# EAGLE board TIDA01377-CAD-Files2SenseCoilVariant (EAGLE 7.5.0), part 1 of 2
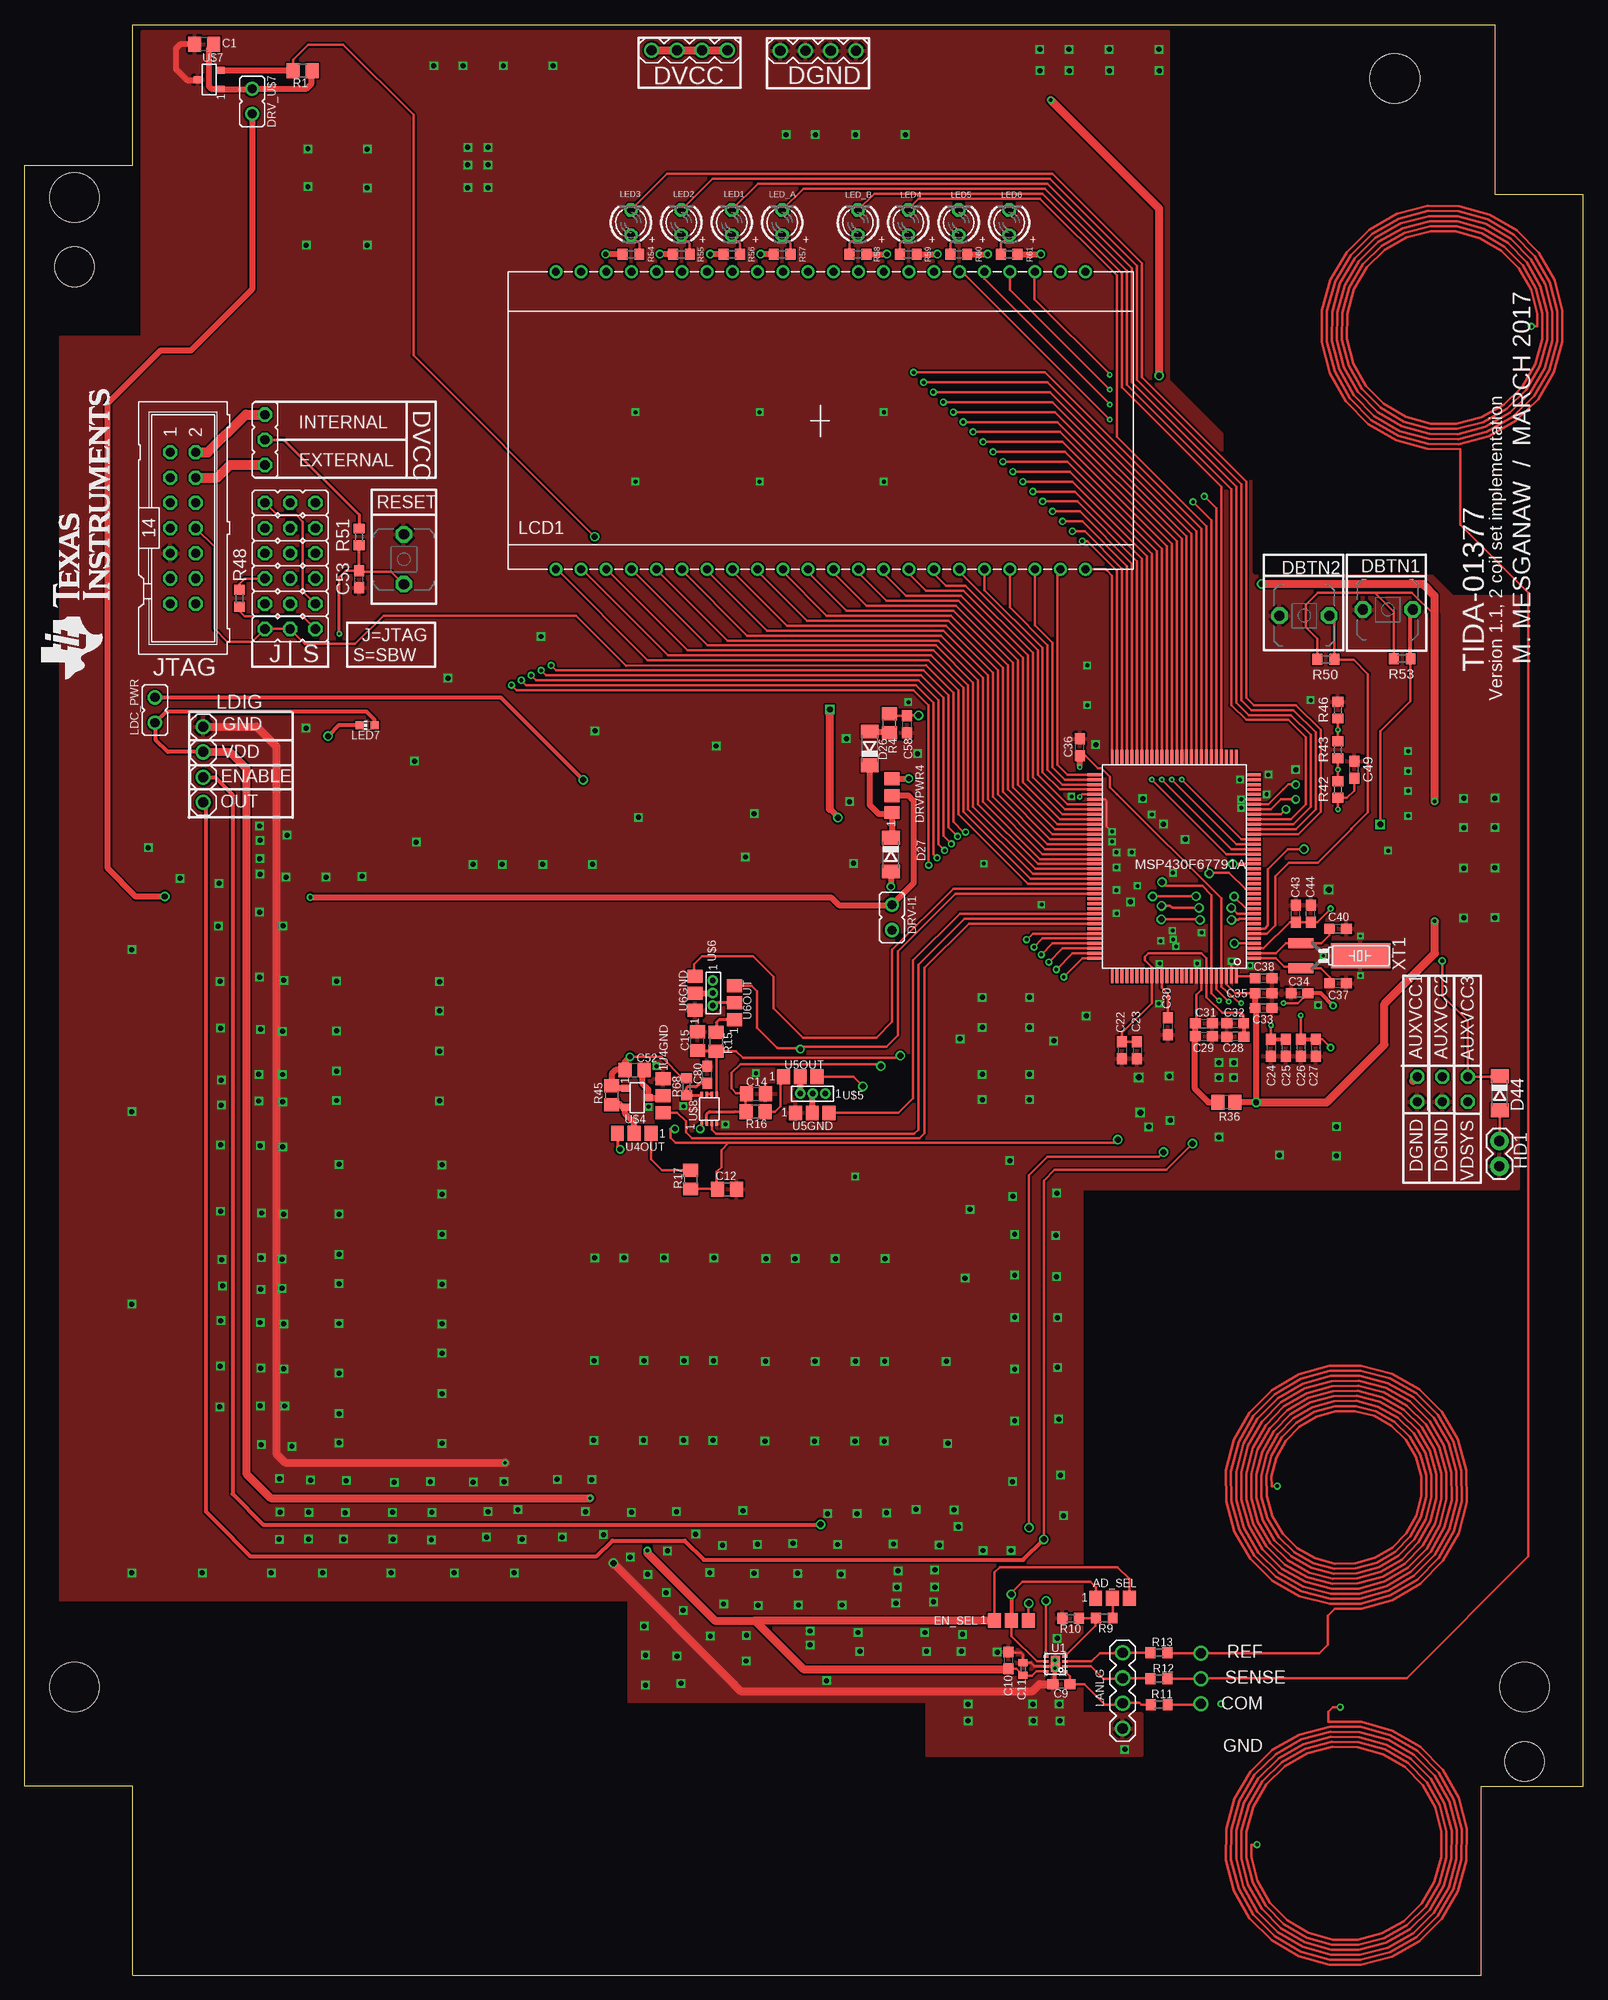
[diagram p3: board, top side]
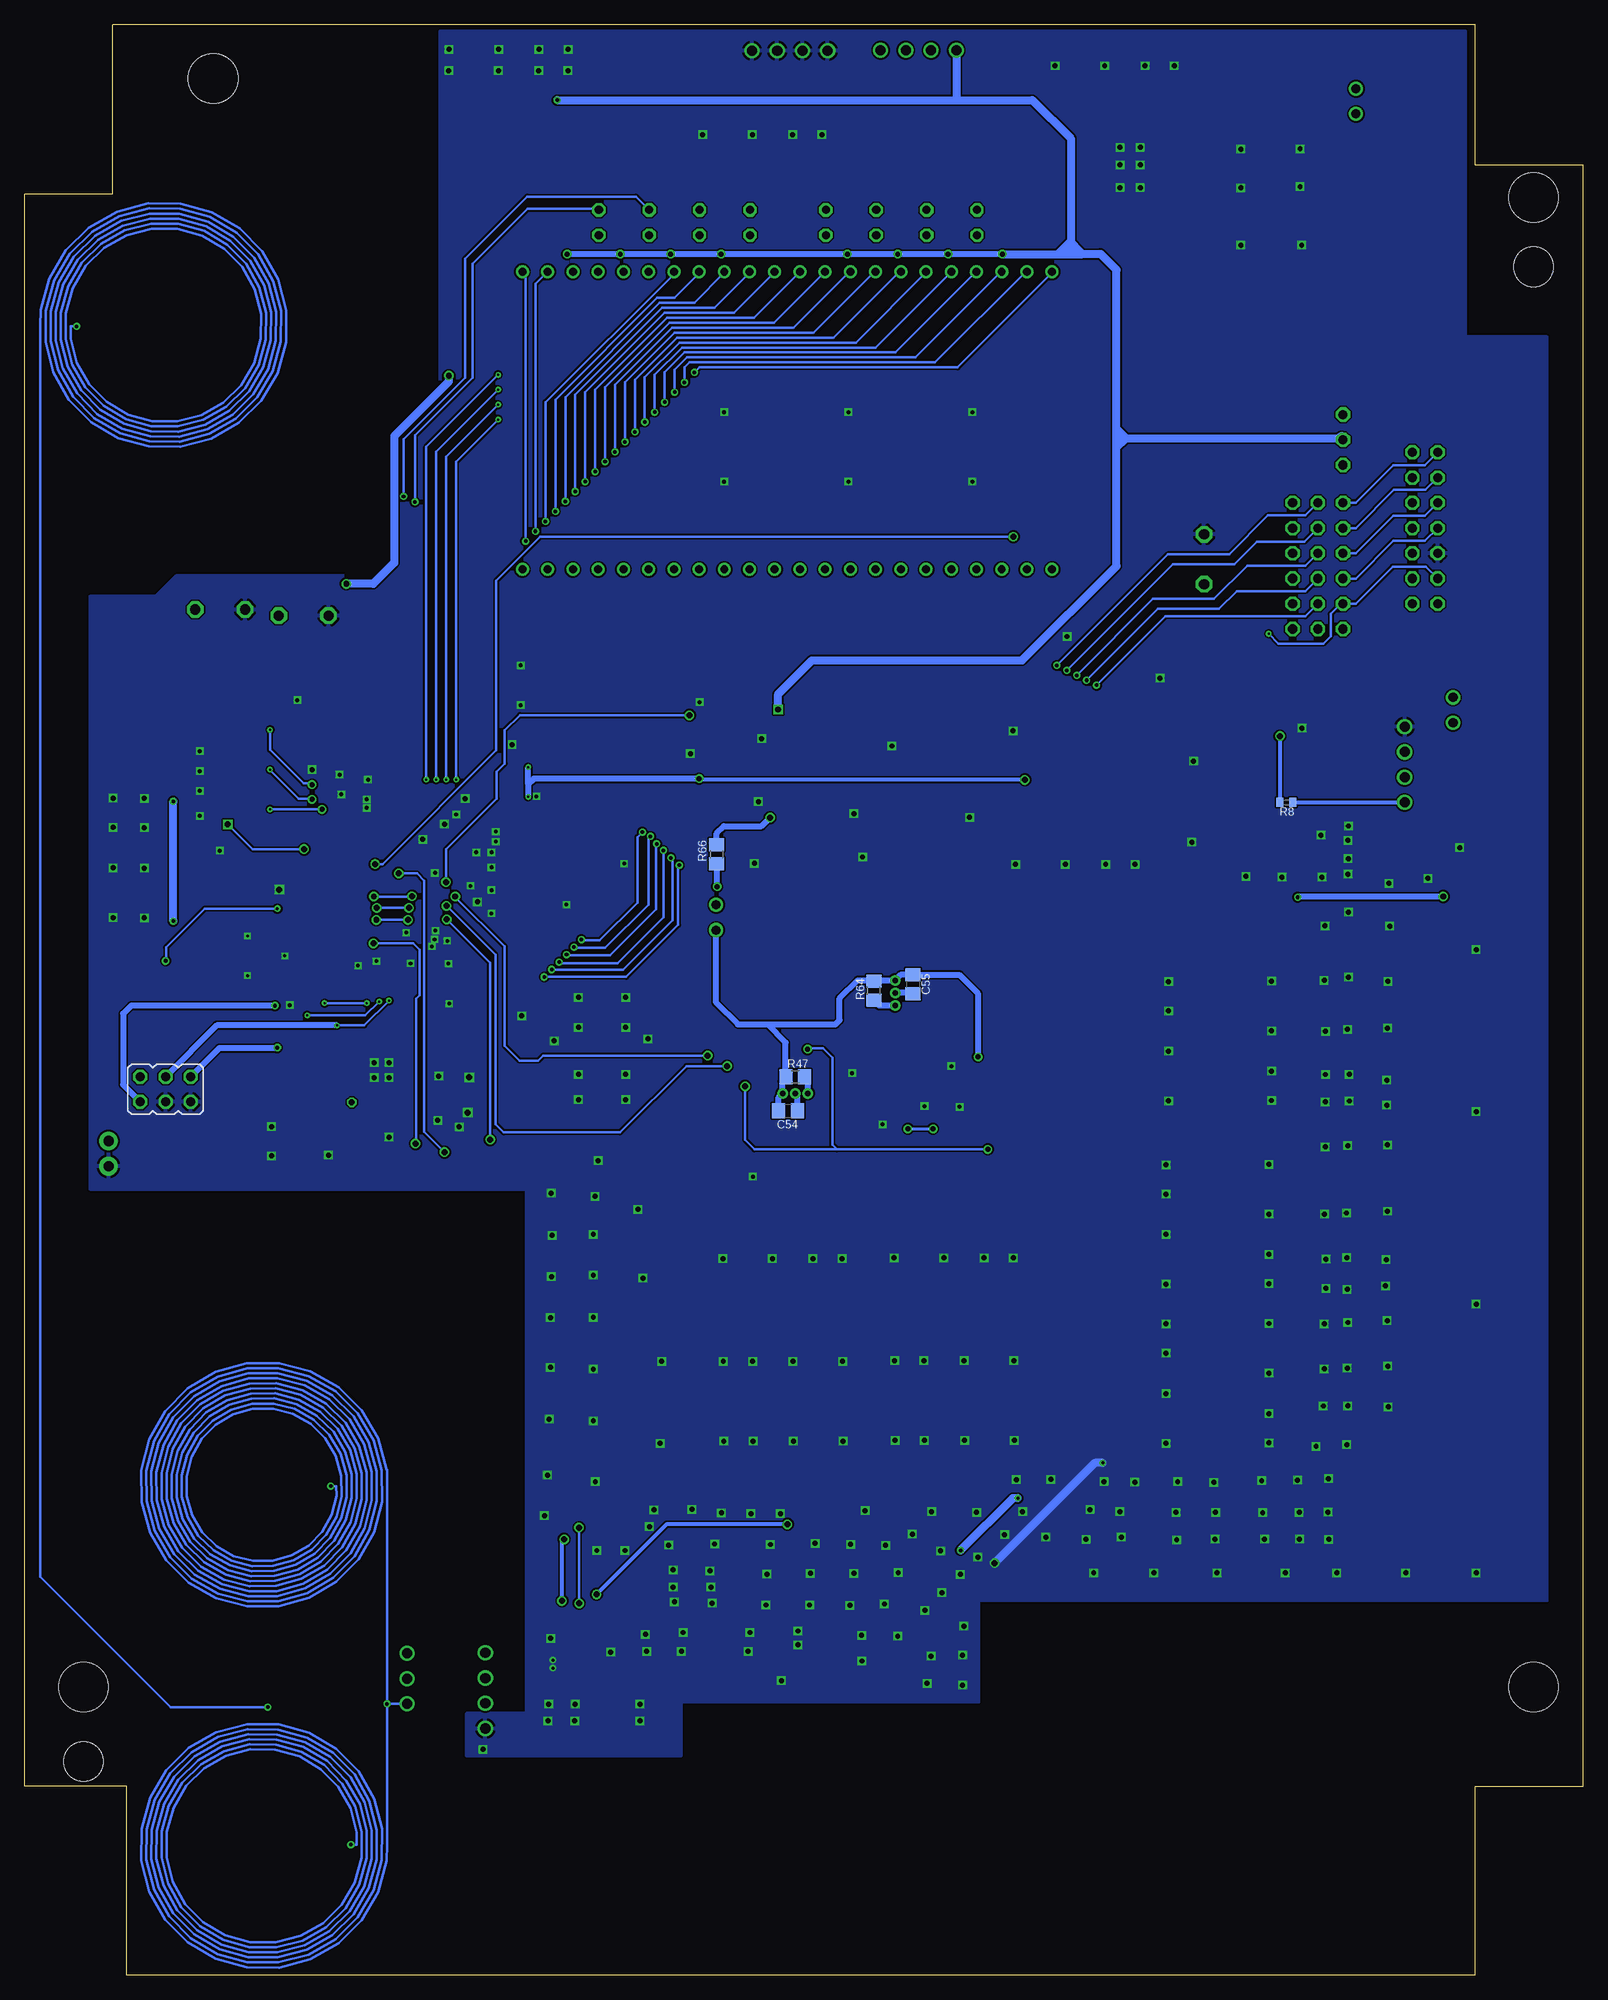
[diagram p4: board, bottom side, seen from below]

Size 156.94 x 196.36 mm. Coordinates in mm from the lower left corner, seen from the top.
Outline: 146.68,0 146.68,19 156.94,19 156.94,179.29 148.1,179.29 148.1,196.36 10.88,196.36 10.88,182.2 0,182.2 0,19 10.88,19 10.88,0 146.68,0
Copper layers (1*16): Top 0.0356mm / dielectric 1.5011mm / Bottom 0.0356mm
Design rules "SilverCircuits *": minimum track width 7mil, minimum drill 7.5mil, track to track 7mil, track to pad 7mil, pad to pad 7mil, via to via 7mil, smd to smd 0mil, copper to edge 20mil, drill to drill 8mil, minimum pad ring 10mil, minimum via ring 7mil, stop-mask expansion 4mil, vias tented up to drill 17mil, thermal gap 10mil
Holes 5 mm at 137.97,190.95 5,178.99 5,29 151.04,29
Holes 4 mm at 5,172 151.04,21.5

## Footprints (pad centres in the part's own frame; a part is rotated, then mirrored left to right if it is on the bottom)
A0R-JMP = smd 1.5 x 1.3: 1 0,1.7; 2 0,0; 3 0,-1.7
C0805 = smd 1.3 x 1.5: 1 -0.95,0; 2 0.95,0
C0603 = smd 1.1 x 1: 1 -0.85,0; 2 0.85,0
C0402 = smd 0.7 x 0.9: 1 -0.65,0; 2 0.65,0
SOD80C = smd 1.4 x 1.8: A 1.7,0; C -1.7,0
PBTH = drill 1.016 pad 1.676 octagon: 1 -0.001,0.001; 2 5.001,0.001
MA04-1 = drill 1.016: 1 -3.81,0; 2 -1.27,0; 3 1.27,0; 4 3.81,0
JP1 = drill 0.914: 1 0,-1.27; 2 0,1.27
1X02 = drill 1.016 pad 1.88: 1 0,0; 2 2.54,0
JP2 = drill 0.914 octagon: 1 -2.54,0; 2 0,0; 3 2.54,0
ML14 = drill 0.914 octagon: 1 -7.62,-1.27; 2 -7.62,1.27; 3 -5.08,-1.27; 4 -5.08,1.27; 5 -2.54,-1.27; 6 -2.54,1.27; 7 0,-1.27; 8 0,1.27; 9 2.54,-1.27; 10 2.54,1.27; 11 5.08,-1.27; 12 5.08,1.27; 13 7.62,-1.27; 14 7.62,1.27
TI_160SEG_LCD = drill 0.8: 1 4.826,0; 2 7.366,0; 3 9.906,0; 4 12.446,0; 5 14.986,0; 6 17.526,0; 7 20.066,0; 8 22.606,0; 9 25.146,0; 10 27.686,0; 11 30.226,0; 12 32.766,0; 13 35.306,0; 14 37.846,0; 15 40.386,0; 16 42.926,0; 17 45.466,0; 18 48.006,0; 19 50.546,0; 20 53.086,0; 21 55.626,0; 22 58.166,0; 23 58.166,29.972; 24 55.626,29.972; 29 42.926,29.972; 30 40.386,29.972; 31 37.846,29.972; 32 35.306,29.972; 33 32.766,29.972; 34 30.226,29.972; 35 27.686,29.972; 36 25.146,29.972; 37 22.606,29.972; 38 20.066,29.972; 39 17.526,29.972; 40 14.986,29.972; 41 12.446,29.972; 42 9.906,29.972; 43 7.366,29.972; 44 4.826,29.972; COM0 45.466,29.972; COM1 48.006,29.972; COM2 50.546,29.972; COM3 53.086,29.972
LED3MM = drill 0.813 octagon: A -1.27,0; K 1.27,0
CHIP-LED0603 = smd 0.8 x 0.8: A 0,-0.75; C 0,0.75
PEU128 = smd 0.3 x 1.4: 1 -9,-7.8; 2 -8.5,-7.8; 3 -8,-7.8; 4 -7.5,-7.8; 5 -7,-7.8; 6 -6.5,-7.8; 7 -6,-7.8; 8 -5.5,-7.8; 9 -5,-7.8; 10 -4.5,-7.8; 11 -4,-7.8; 12 -3.5,-7.8; 13 -3,-7.8; 14 -2.5,-7.8; 15 -2,-7.8; 16 -1.5,-7.8; 17 -1,-7.8; 18 -0.5,-7.8; 19 0,-7.8; 20 0.5,-7.8; 21 1,-7.8; 22 1.5,-7.8; 23 2,-7.8; 24 2.5,-7.8; 25 3,-7.8; 26 3.5,-7.8; 27 4,-7.8; 28 4.5,-7.8; 29 5,-7.8; 30 5.5,-7.8; 31 6,-7.8; 32 6.5,-7.8; 33 7,-7.8; 34 7.5,-7.8; 35 8,-7.8; 36 8.5,-7.8; 37 9,-7.8; 38 9.5,-7.8; 65 9.5,8.3; 66 9,8.3; 67 8.5,8.3; 68 8,8.3; 69 7.5,8.3; 70 7,8.3; 71 6.5,8.3; 72 6,8.3; 73 5.5,8.3; 74 5,8.3; 75 4.5,8.3; 76 4,8.3; 77 3.5,8.3; 78 3,8.3; 79 2.5,8.3; 80 2,8.3; 81 1.5,8.3; 82 1,8.3; 83 0.5,8.3; 84 0,8.3; 85 -0.5,8.3; 86 -1,8.3; 87 -1.5,8.3; 88 -2,8.3; 89 -2.5,8.3; 90 -3,8.3; 91 -3.5,8.3; 92 -4,8.3; 93 -4.5,8.3; 94 -5,8.3; 95 -5.5,8.3; 96 -6,8.3; 97 -6.5,8.3; 98 -7,8.3; 99 -7.5,8.3; 100 -8,8.3; 101 -8.5,8.3; 102 -9,8.3 | smd 1.4 x 0.3: 39 11.3,-6; 40 11.3,-5.5; 41 11.3,-5; 42 11.3,-4.5; 43 11.3,-4; 44 11.3,-3.5; 45 11.3,-3; 46 11.3,-2.5; 47 11.3,-2; 48 11.3,-1.5; 49 11.3,-1; 50 11.3,-0.5; 51 11.3,0; 52 11.3,0.5; 53 11.3,1; 54 11.3,1.5; 55 11.3,2; 56 11.3,2.5; 57 11.3,3; 58 11.3,3.5; 59 11.3,4; 60 11.3,4.5; 61 11.3,5; 62 11.3,5.5; 63 11.3,6; 64 11.3,6.5; 103 -10.8,6.5; 104 -10.8,6; 105 -10.8,5.5; 106 -10.8,5; 107 -10.8,4.5; 108 -10.8,4; 109 -10.8,3.5; 110 -10.8,3; 111 -10.8,2.5; 112 -10.8,2; 113 -10.8,1.5; 114 -10.8,1; 115 -10.8,0.5; 116 -10.8,0; 117 -10.8,-0.5; 118 -10.8,-1; 119 -10.8,-1.5; 120 -10.8,-2; 121 -10.8,-2.5; 122 -10.8,-3; 123 -10.8,-3.5; 124 -10.8,-4; 125 -10.8,-4.5; 126 -10.8,-5; 127 -10.8,-5.5; 128 -10.8,-6
R0805 = smd 1.3 x 1.5: 1 -0.95,0; 2 0.95,0
R0402 = smd 0.7 x 0.9: 1 -0.65,0; 2 0.65,0
R0603 = smd 1 x 1.1: 1 -0.85,0; 2 0.85,0
R0805' = smd 1.3 x 1.5: 1 -0.85,0; 2 0.85,0
JP3Q = drill 0.914 octagon: 1 -2.54,-1.27; 2 -2.54,1.27; 3 0,-1.27; 4 0,1.27; 5 2.54,-1.27; 6 2.54,1.27
DSG0008A = smd 0.508 x 0.254: 1 -0.95,0.75; 2 -0.95,0.25; 3 -0.95,-0.25; 4 -0.95,-0.75; 5 0.95,-0.75; 6 0.95,-0.25; 7 0.95,0.25; 8 0.95,0.75 | smd 0.889 x 1.6: 9 0,0
SOT23 = smd 0.7 x 0.8: 1 -0.92,-2.07; 2 0.98,-2.07; 3 0.03,0.275
SIP = drill 0.55: 1 0,0; 2 1.27,0; 3 2.54,0
DCU = smd 0.5 x 0.25: 1 1.39,-0.95; 2 1.39,-1.45; 3 1.39,-1.95; 4 1.39,-2.45; 5 4.29,-2.45; 6 4.29,-1.95; 7 4.29,-1.45; 8 4.29,-0.95
CM200T = smd 1 x 2.5: P1 -1.25,-5; P2 1.25,-5 | smd 2.5 x 6: P3 0,1

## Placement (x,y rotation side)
AD_SEL  0R-JUMPA  [A0R-JMP]  109.55,37.96 270 top
C1  DNP  [C0805]  18.06,194.4 180 top
C9  27pF  [C0603]  104.39,29.3 180 top
C10  1u  [C0603]  99.08,31.69 90 top
C11  0.1u  [C0402]  100.53,30.83 90 top
C12  DNP  [C0805]  70.71,79.14 0 top
C14  DNP  [C0805]  73.63,88.74 0 top
C15  DNP  [C0805]  67.74,94.05 90 top
C22  4.7uF  [C0603]  110.51,93.12 270 top
C23  100nF  [C0603]  112.01,93.12 270 top
C24  4.7uF  [C0603]  125.51,93.38 270 top
C25  100nF  [C0603]  127.01,93.38 270 top
C26  4.7uF  [C0603]  128.51,93.38 270 top
C27  100nF  [C0603]  130.01,93.38 270 top
C28  100nF  [C0603]  121.91,94.5 180 top
C29  4.7uF  [C0603]  118.76,94.53 0 top
C30  100nF  [C0603]  115.11,95.53 270 top
C31  100nF  [C0603]  118.76,95.83 0 top
C32  4.7uF  [C0603]  121.9,95.83 180 top
C33  100nF  [C0603]  124.76,97.38 0 top
C34  4.7uF  [C0603]  128.38,98.88 180 top
C35  4.7uF  [C0603]  124.76,98.88 0 top
C36  100nF  [C0603]  106.26,123.62 90 top
C37  12pF  [C0603]  132.26,99.88 0 top
C38  0.47uF  [C0603]  124.76,100.38 0 top
C40  12pF  [C0603]  132.26,105.38 0 top
C43  100nF  [C0603]  128.01,106.88 90 top
C44  0.47uF  [C0603]  129.51,106.88 90 top
C49  4.7uF  [C0603]  133.88,121.38 90 top
C52  DNP  [C0805]  61.4,91.14 0 top
C53  0.1uF  [C0603]  33.67,140.56 90 top
C54  DNP  [C0805]  80.08,87.02 0 bottom
C55  DNP  [C0805]  67.51,99.77 270 bottom
C58  DNP  [C0603]  88.82,125.95 270 top
C80  DNP  [C0603]  68.73,90.67 90 top
D26  PMLL4148  [SOD80C]  85.09,123.51 90 top
D27  PMLL4148  [SOD80C]  87.22,112.82 270 top
D44  [SOD80C]  148.54,88.79 270 top
DBTN1  [PBTH]  134.77,137.49 0 top
DBTN2  [PBTH]  126.36,136.88 0 top
DGND  [MA04-1]  79.9,193.75 0 top
DRV-I1  [JP1]  87.32,106.49 0 top
DRV_U$7  [JP1]  22.88,188.66 180 top
DRVPWR4  0R-JUMPA  [A0R-JMP]  87.32,118.76 0 top
DVCC  [MA04-1]  66.94,193.8 0 top
EN_SEL  0R-JUMPA  [A0R-JMP]  99.36,35.7 270 top
HD1  [1X02]  148.51,81.45 90 top
JP4  [JP2]  26.72,135.54 180 top
JP5  [JP2]  26.72,138.08 180 top
JP6  [JP2]  26.72,140.62 180 top
JP7  [JP2]  26.72,143.16 180 top
JP8  [JP2]  26.72,145.7 180 top
JP9  [JP2]  26.72,148.24 180 top
JP10  [JP2]  24.18,154.59 270 top
JTAG  [ML14]  15.93,145.7 270 top
LANLG  [MA04-1]  110.56,28.64 90 top
LCD1  TI_160SEG_LCD  [TI_160SEG_LCD]  48.65,141.53 0 top
LDC_PWR  [JP1]  13.1,127.37 0 top
LDIG  [MA04-1]  17.98,121.89 90 top
LED1  [LED3MM]  71.2,176.46 90 top
LED2  [LED3MM]  66.12,176.46 90 top
LED3  [LED3MM]  61.04,176.46 90 top
LED4  [LED3MM]  88.98,176.46 90 top
LED5  [LED3MM]  94.06,176.46 90 top
LED6  [LED3MM]  99.14,176.46 90 top
LED7  [CHIP-LED0603]  34.47,125.85 90 top
LED_A  [LED3MM]  76.28,176.46 90 top
LED_B  [LED3MM]  83.9,176.46 90 top
MSP430F67791A  MSP430F6779AIPEU  [PEU128]  116.01,111.38 90 top
R1  DNP  [R0805]  27.99,191.74 180 top
R4  DNP  [R0805]  87.07,126.05 90 top
R8  200  [R0402]  29.89,118.08 180 bottom
R9  49.9k  [R0603]  108.71,35.96 0 top
R10  9.31k(One Sense Coil); 44.2k(Two Sense Coil)  [R0603]  105.33,35.93 0 top
R11  0  [R0603]  114.25,27.25 0 top
R12  0  [R0603]  114.22,29.84 0 top
R13  0  [R0603]  114.22,32.48 0 top
R15  DNP  [R0805]  69.62,93.97 90 top
R16  DNP  [R0805]  73.58,86.94 0 top
R17  DNP  [R0805]  67.05,80.1 90 top
R36  10R  [R0805']  121.02,87.89 180 top
R42  560k  [R0603]  132.26,119.38 270 top
R43  560k  [R0603]  132.26,123.38 270 top
R45  DNP  [R0805]  59.11,88.58 270 top
R46  560k  [R0603]  132.26,127.38 270 top
R47  DNP  [R0805]  79.35,90.45 0 bottom
R48  330  [R0603]  21.62,138.62 270 top
R50  100K  [R0603]  131.04,132.48 0 top
R51  47K  [R0603]  33.67,144.81 270 top
R53  100K  [R0603]  138.71,132.53 0 top
R54  100  [R0603]  61.04,173.28 0 top
R55  100  [R0603]  66.12,173.28 0 top
R56  100  [R0603]  71.2,173.28 0 top
R57  100  [R0603]  76.28,173.28 0 top
R58  100  [R0603]  83.9,173.28 180 top
R59  100  [R0603]  88.98,173.28 180 top
R60  100  [R0603]  94.06,173.28 180 top
R61  100  [R0603]  99.14,173.28 180 top
R64  DNP  [R0805]  71.44,99.11 270 bottom
R66  DNP  [R0805]  87.27,112.87 90 bottom
R68  DNP  [R0603]  66.62,89.45 90 top
RESET  [PBTH]  38.17,140.06 90 top
SV1  [JP3Q]  142.77,89.2 0 bottom
U1  Value  [DSG0008A]  103.78,31.34 180 top
U4GND  0R-JUMPA  [A0R-JMP]  64.29,88.54 180 top
U4OUT  0R-JUMPA  [A0R-JMP]  61.37,84.78 90 top
U5GND  0R-JUMPA  [A0R-JMP]  79.31,86.81 270 top
U5OUT  0R-JUMPA  [A0R-JMP]  78.09,90.44 270 top
U6GND  0R-JUMPA  [A0R-JMP]  67.51,98.86 0 top
U6OUT  0R-JUMPA  [A0R-JMP]  71.48,97.9 0 top
U$4  DRV5033_SOT23  [SOT23]  62.53,88.38 270 top
U$5  DRV5033_SIP  [SIP]  80.62,88.78 180 top
U$6  DRV5033_SIP  [SIP]  69.29,100.16 270 top
U$7  DRV5033_SOT23  [SOT23]  17.68,190.82 90 top
U$8  SN74AUP2G32  [DCU]  67.23,84.38 90 top
XT1  [CM200T]  133.51,102.62 270 top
